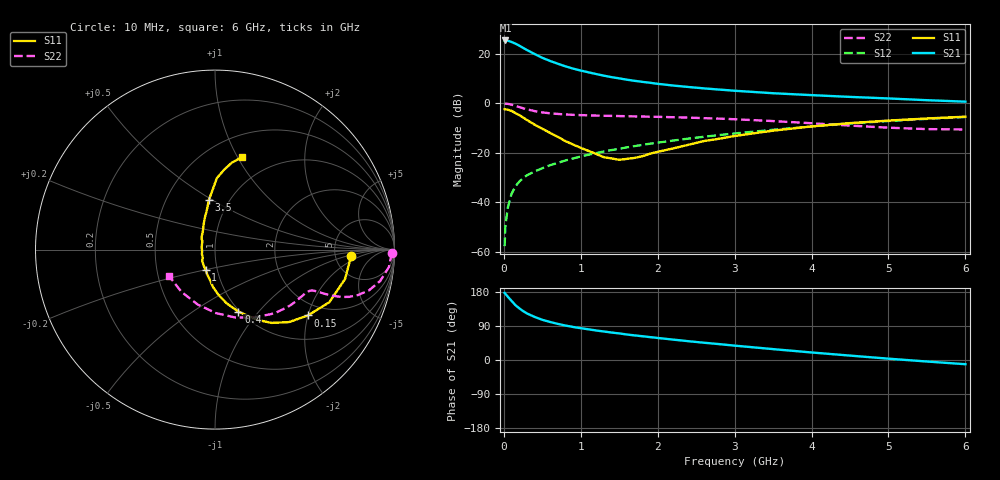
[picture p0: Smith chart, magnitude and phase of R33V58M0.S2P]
! SIEMENS Small Signal Semiconductors
! BFR181
! Si NPN RF Bipolar Junction Transistor in SOT23
! VCE = 3.5 V  IC = 8 mA
! Common Emitter S-Parameters:  May  1996
# GHz  S  MA  R  50
!  f  S11  S21  S12  S22
! GHz  MAG  ANG  MAG  ANG  MAG  ANG  MAG  ANG
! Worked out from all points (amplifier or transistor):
!   36 points, 10 MHz to 6 GHz, reference 50 ohm
!   highest |S21| = 25.4 dB at 20 MHz (marker M1)
!   |S21| within 3 dB of that: start of sweep to 250.6 MHz
!   unconditionally stable (mu >= 1): 872.8 MHz to 2.732 GHz
!   at 250 MHz: K = 0.54, MSG = 26.3 dB, |S12| = -30.2 dB
!   at 1.4 GHz: K = 1.06, MAG = 13.3 dB, |S12| = -18.9 dB
!   at 6 GHz: K = 0.86, MSG = 3.1 dB, |S12| = -5.6 dB
!   S11 on the Smith chart (normalised r, x): 10 MHz: 7.09, -1.20; 150 MHz: 1.63, -2.00; 400 MHz: 0.99, -0.79; 1 GHz: 0.88, -0.21; 3.5 GHz: 0.80, +0.48; 6 GHz: 0.72, +1.04
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0.01  0.7589 -2.7  18.54 177.1  0.0013 86.9  0.9874 -1.1
0.02  0.7532 -5.1  18.55 174.6  0.0033 85.0  0.981 -2.4
0.05  0.743 -12.7  18.36 167.4  0.0076 86.3  0.974 -5.7
0.1  0.7013 -24.7  17.3 156.1  0.0148 76.7  0.9366 -10.8
0.15  0.6347 -35.3  16.02 144.8  0.0209 73.1  0.8878 -14.8
0.2  0.5772 -44.4  14.58 136.5  0.0261 70.8  0.8366 -17.6
0.25  0.5162 -52.3  13.14 129.1  0.0308 68.9  0.7928 -19.4
0.3  0.4591 -58.7  11.9 122.9  0.0351 68.3  0.7543 -20.5
0.4  0.3699 -69.3  9.876 113.7  0.042 66.8  0.6946 -21.6
0.5  0.3053 -77.9  8.263 106.1  0.0487 67.0  0.6539 -22.0
0.6  0.2527 -85.6  7.16 100.4  0.0561 67.2  0.6272 -22.2
0.7  0.2101 -92.8  6.294 95.4  0.0625 67.7  0.6087 -22.4
0.8  0.1721 -99.4  5.571 91.0  0.0699 67.6  0.5948 -22.6
1  0.1257 -114.1  4.573 83.9  0.0839 68.4  0.576 -23.5
1.1  0.1092 -125.3  4.214 81.0  0.0913 68.4  0.5695 -24.2
1.3  0.0813 -147.4  3.605 75.2  0.1061 68.2  0.5593 -25.8
1.6  0.0753 169.8  2.991 67.3  0.1285 67.4  0.5473 -28.7
2.2  0.1223 123.6  2.28 53.8  0.1765 64.8  0.5226 -36.3
3.5  0.2795 97.0  1.594 28.7  0.2914 54.7  0.437 -59.8
4.5  0.3974 88.6  1.344 11.6  0.3889 43.9  0.3537 -89.2
5.5  0.4928 79.1  1.153 -4.0  0.4834 31.1  0.3006 -128.5
6  0.536 73.9  1.077 -11.1  0.5267 24.1  0.2955 -150.4
